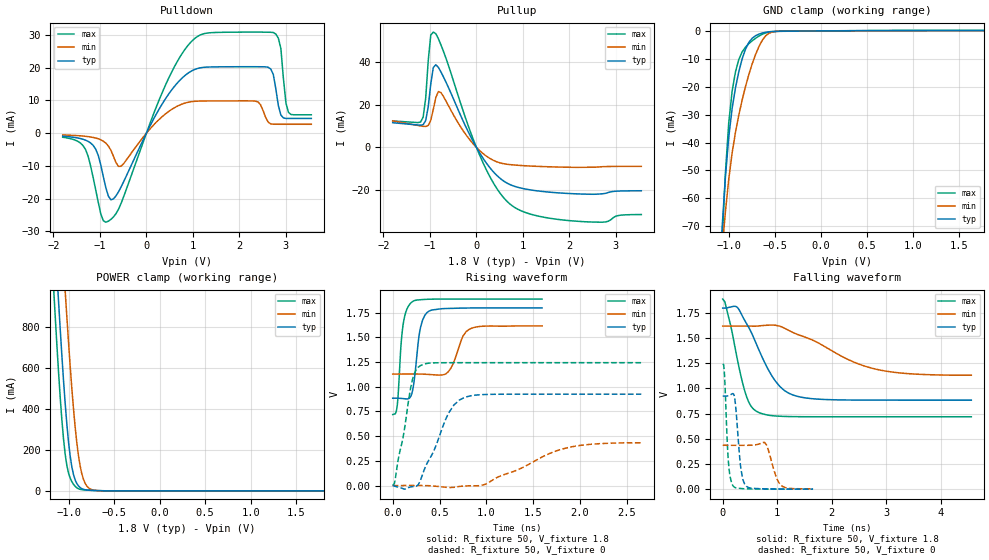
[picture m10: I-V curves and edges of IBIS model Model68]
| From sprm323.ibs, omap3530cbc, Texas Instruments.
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| Model based on original model for BQ0226CS_7LM
|   Sub model BQ0226CS_7LM_PD_ON_1P8
[model]   Model68
|[Input Load]   PD
|[Output Drive]
|Voltage   1.8V
|Mode   I/O
Model_type   I/O
Polarity   Non-Inverting
Enable   Active-Low
Vinl =  0.63
Vinh =  1.17
Cref =  15.0000pF
Rref =  100.0000M
Vref =  0V
Vmeas =  0.9
C_comp   0.742316p   0.619633p   0.9008309p
[Model Spec]
Vinl   0.63   0.567   0.6615
Vinh   1.17   1.053   1.2285
[Temperature Range]   25   125   -40
[Voltage Range]   1.8   1.62   1.89
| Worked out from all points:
|   slope of the pulldown table from 0 to 0.27 V, typ, clamps not added: 37.2 ohm
|   slope of the pullup table from 0 to 0.27 V, typ, clamps not added: 30.1 ohm
|   GND clamp passes 1 mA (typ) near -0.66 V on its own axis
|   POWER clamp passes 1 mA (typ) near -0.62 V on its own axis
|   rising waveform, R_fixture 50, V_fixture 1.8: 20-80 % time 71.4ps typ, 114ps min, 55.3ps max; typ from 0.884 V to 1.8 V
|   rising waveform, R_fixture 50, V_fixture 0: 20-80 % time 254ps typ, 609ps min, 137ps max; typ from 0 V to 0.925 V
|   falling waveform, R_fixture 50, V_fixture 1.8: 20-80 % time 509ps typ, 1.12ns min, 285ps max; typ from 1.8 V to 0.883 V
|   falling waveform, R_fixture 50, V_fixture 0: 20-80 % time 88.1ps typ, 148ps min, 63.1ps max; typ from 0.925 V to 0 V
[POWER_clamp]
-1.8V     6.299A     6.506A     6.196A
-1.164V   1.344A     1.893A     994.1mA
-1.127V   1.063A     1.63A      711.8mA
-1.109V   925.8mA    1.498A     579.2mA
-1.073V   661.6mA    1.236A     346.9mA
-1.036V   426.8mA    976.8mA    179.1mA
-981.8mV  170.9mA    611.1mA    62.76mA
-909.1mV  36.26mA    236.5mA    15.53mA
-872.7mV  16.5mA     123mA      7.955mA
-836.4mV  7.93mA     57.21mA    5.238mA
-727.3mV  2.341mA    4.355mA    2.385mA
1.8V      125.3uA    51.97uA    219uA
[Pulldown]
-1.8V     -923.4uA   -546.6uA   -1.251mA
-1.364V   -1.871mA   -894.2uA   -3.779mA
-1.145V   -3.734mA   -1.313mA   -13.56mA
-818.2mV  -19.23mA   -3.925mA   -26.88mA
-545.5mV  -16.45mA   -10.11mA   -21.46mA
600mV     14.23mA    7.738mA    20.23mA
1.364V    20.2mA     9.834mA    30.64mA
2.618V    20.12mA    3.366mA    30.81mA
2.782V    13.57mA    2.716mA    30.26mA
2.891V    5.527mA    2.714mA    25.86mA
3.055V    4.494mA    2.712mA    6.327mA
3.545V    4.488mA    2.709mA    5.61mA
[Pullup]
-1.8V     11.56mA    12.44mA    12.38mA
-1.145V   10.65mA    9.865mA    14.2mA
-1.091V   12.57mA    9.798mA    23mA
-1.036V   19.01mA    10.29mA    40.58mA
-981.8mV  29.64mA    12.69mA    52.61mA
-927.3mV  37.42mA    17.78mA    54mA
-818.2mV  37.48mA    26.16mA    50.92mA
-763.6mV  35.38mA    25.7mA     48.06mA
54.55mV   -2.036mA   -1.184mA   -2.864mA
709.1mV   -17.28mA   -8.025mA   -26.29mA
2.073V    -21.67mA   -9.32mA    -34.42mA
3.545V    -20.3mA    -8.865mA   -31.43mA
[GND_clamp]
-1.8V     -645.6mA   -500mA     -849.8mA
-1.073V   -71.08mA   -78.89mA   -76.42mA
-1.036V   -52.54mA   -64.93mA   -51.21mA
-1V       -38.13mA   -53.23mA   -32.98mA
-963.6mV  -27.9mA    -43.88mA   -21.73mA
-927.3mV  -20.45mA   -36.39mA   -14.71mA
-890.9mV  -14.64mA   -30.18mA   -10.24mA
-818.2mV  -6.518mA   -19.93mA   -5.792mA
-709.1mV  -1.723mA   -8.439mA   -2.636mA
-600mV    -489.4uA   -1.77mA    -731.6uA
-490.9mV  -149.5uA   -195.2uA   -195.1uA
1.764V    125uA      52.51uA    217.2uA
[Ramp]
dV/dt_f  0.5592749/0.5182849n   0.300643/1.16002n   0.7140734/0.2899365n
dV/dt_r  0.5767956/0.2621776n  0.2745133/0.6380198n  0.7741709/0.1410793n
R_load = 50
[Rising Waveform]
R_fixture = 50
V_fixture = 1.8
V_fixture_min = 1.62
V_fixture_max = 1.89
0s        883.5mV    1.128V     718.5mV
48ps      883.6mV    1.128V     807.6mV
90ps      881.7mV    1.128V     1.438V
112ps     879.8mV    1.128V     1.633V
204ps     928.6mV    1.129V     1.856V
298ps     1.604V     1.128V     1.88V
388ps     1.765V     1.124V     1.885V
594ps     1.792V     1.151V     1.887V
822ps     1.797V     1.583V     1.887V
1.596ns   1.798V     1.616V     1.887V
[Rising Waveform]
R_fixture = 50
V_fixture = 0
V_fixture_min = 0
V_fixture_max = 0
0s        159.6nV    65.92nV    359nV
18ps      -6.098mV   -2.37uV    21.55mV
110ps     -31.67mV   57.3uV     484.7mV
210ps     -10.91mV   236.5uV    1.069V
312ps     93.83mV    160.8uV    1.221V
598ps     734.2mV    -20.74mV   1.243V
768ps     891.8mV    -4.364mV   1.243V
996ps     921.6mV    14.51mV    1.243V
1.85ns    924.6mV    378.9mV    1.243V
2.656ns   924.6mV    432.5mV    1.243V
[Falling Waveform]
R_fixture = 50
V_fixture = 1.8
V_fixture_min = 1.62
V_fixture_max = 1.89
0s        1.798V     1.619V     1.887V
54ps      1.797V     1.619V     1.828V
258ps     1.809V     1.619V     1.318V
414ps     1.665V     1.619V     958.3mV
526ps     1.554V     1.618V     819.1mV
664ps     1.383V     1.62V      760.5mV
970ps     1.071V     1.627V     726.6mV
1.368ns   921.6mV    1.537V     719.6mV
2.814ns   883.8mV    1.191V     718.5mV
4.562ns   883.5mV    1.131V     718.5mV
[Falling Waveform]
R_fixture = 50
V_fixture = 0
V_fixture_min = 0
V_fixture_max = 0
0s        924.6mV    435.8mV    1.243V
34ps      924mV      435.9mV    1.123V
106ps     927.9mV    435.7mV    262.2mV
186ps     948.8mV    435.4mV    36.01mV
232ps     851.7mV    435.4mV    15.18mV
336ps     193.5mV    435.3mV    6.333mV
436ps     27.96mV    435.4mV    3.331mV
770ps     3.296mV    464.1mV    963.5uV
1.086ns   1.572mV    31.63mV    211.8uV
1.658ns   419.5uV    3.255mV    19.93uV
